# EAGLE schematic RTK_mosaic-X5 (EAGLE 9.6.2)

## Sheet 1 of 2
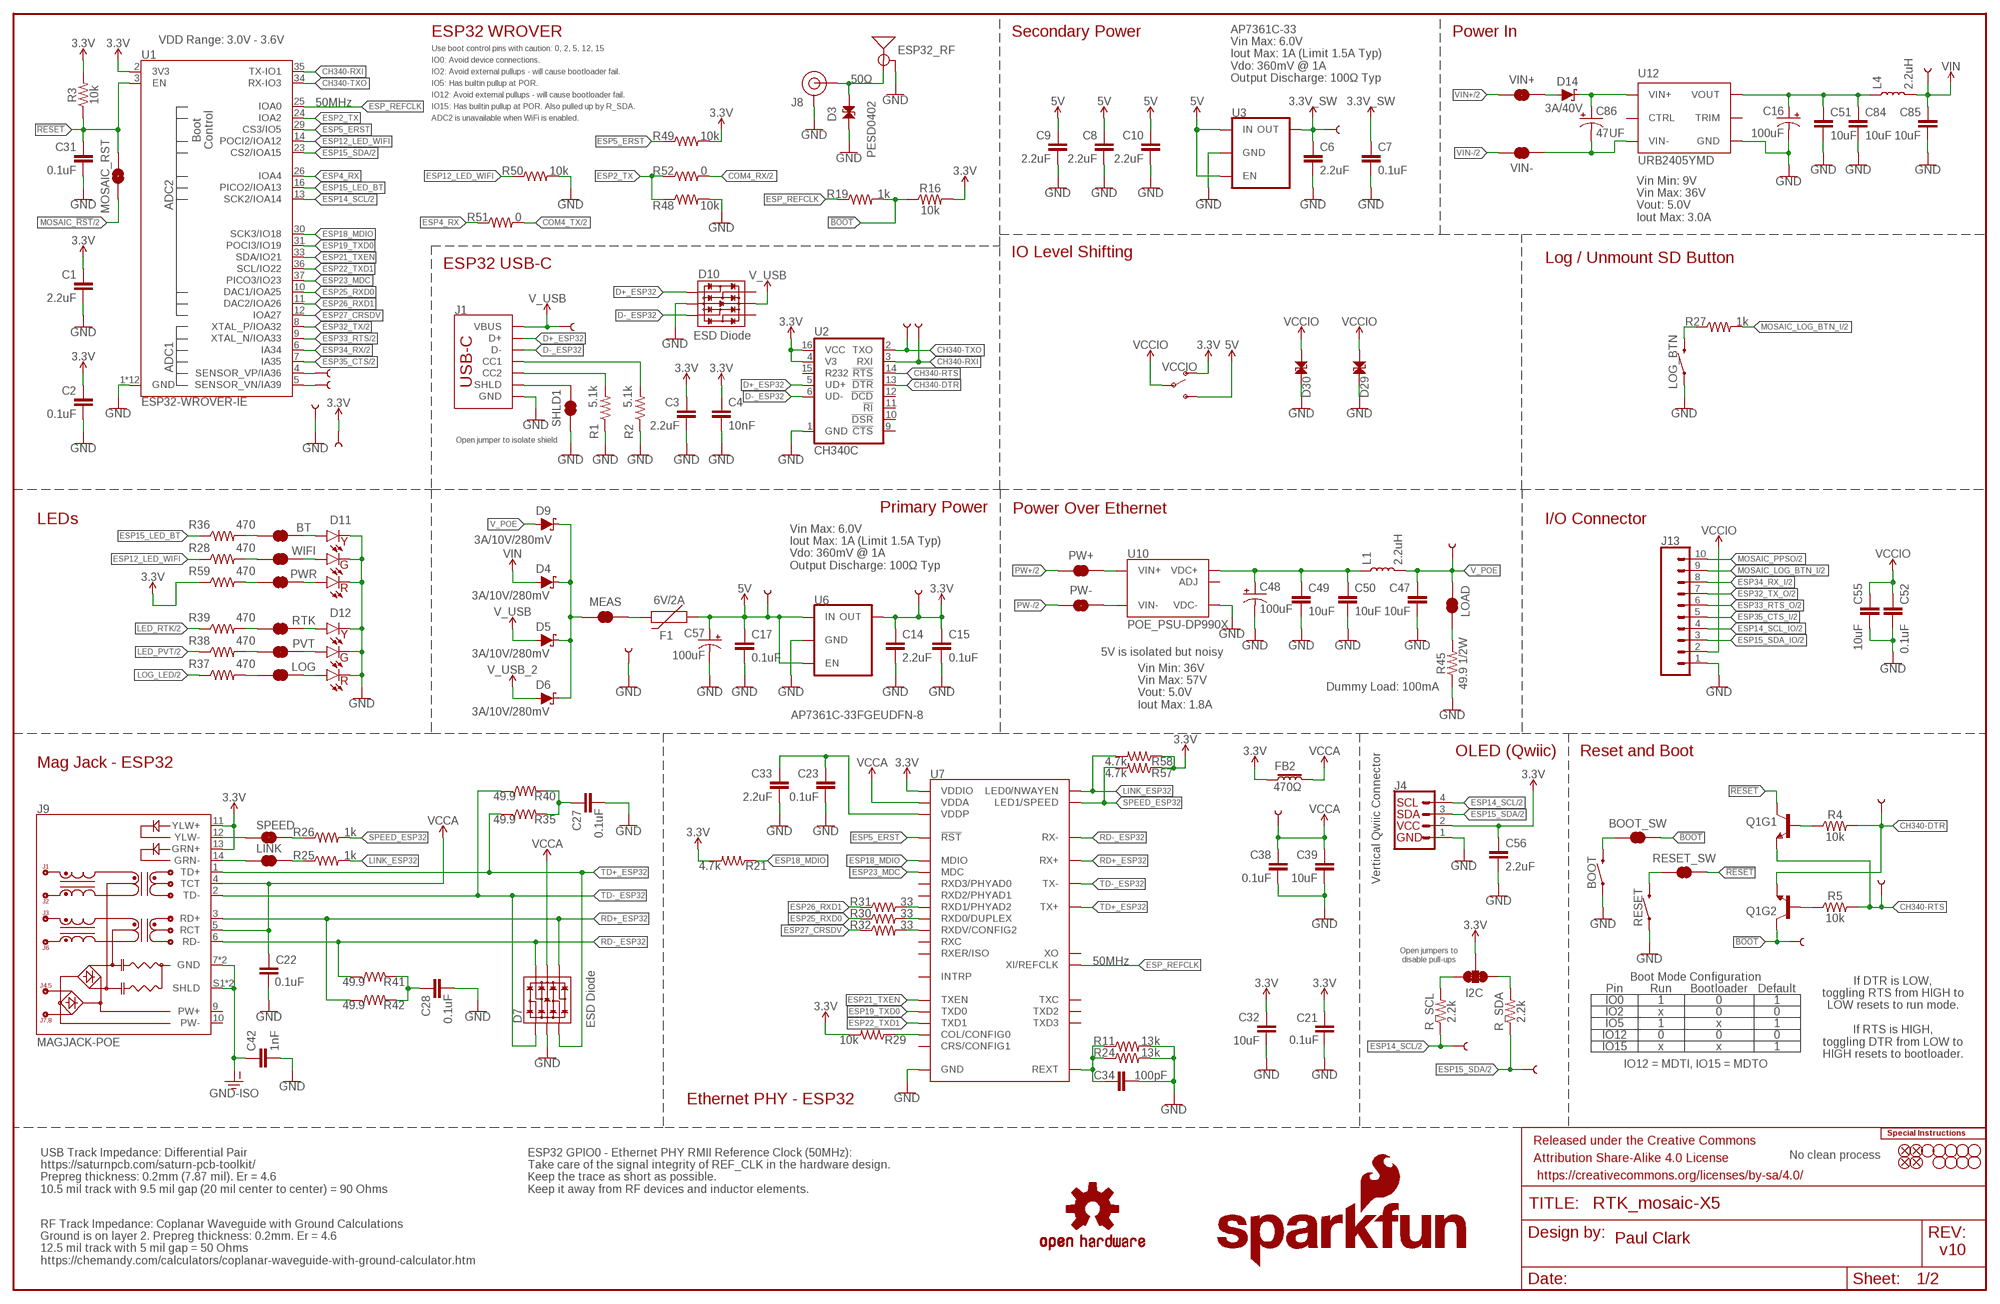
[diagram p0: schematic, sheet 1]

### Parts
3V3  TEST-POINTPOGO_PTH  [1X01_NO_SILK]
3V3_SW  TEST-POINTPOGO_PTH  [1X01_NO_SILK]
5V  TEST-POINTPOGO_PTH  [1X01_NO_SILK]
BOOT  MOMENTARY-SWITCH-SPST-PTH-RIGHT-ANGLE-8-020  [TACTILE_SWITCH_PTH_RA_8-020]
BOOT_SW  JUMPER-SMT_2_NC_TRACE_SILK  [SMT-JUMPER_2_NC_TRACE_SILK]
BT  JUMPER-SMT_2_NC_TRACE_SILK  [SMT-JUMPER_2_NC_TRACE_SILK]
C1  2.2uF  2.2UF-0603-10V-20%  [0603]
C2  0.1uF  0.1UF-0603-25V-5%  [0603]
C3  2.2uF  2.2UF-0603-10V-20%  [0603]
C4  10nF  10NF-0603-50V-10%  [0603]
C6  2.2uF  2.2UF-0603-10V-20%  [0603]
C7  0.1uF  0.1UF-0603-25V-5%  [0603]
C8  2.2uF  2.2UF-0603-10V-20%  [0603]
C9  2.2uF  2.2UF-0603-10V-20%  [0603]
C10  2.2uF  2.2UF-0603-10V-20%  [0603]
C14  2.2uF  2.2UF-0603-10V-20%  [0603]
C15  0.1uF  0.1UF-0603-25V-5%  [0603]
C16  100uF  100UF-POLAR-25V-20%(ELEC)  [PANASONIC_D]
C17  0.1uF  0.1UF-0603-25V-5%  [0603]
C21  0.1uF  0.1UF-0603-25V-5%  [0603]
C22  0.1uF  0.1UF-0603-25V-5%  [0603]
C23  0.1uF  0.1UF-0603-25V-5%  [0603]
C27  0.1uF  0.1UF-0603-25V-5%  [0603]
C28  0.1uF  0.1UF-0603-25V-5%  [0603]
C31  0.1uF  0.1UF-0603-25V-5%  [0603]
C32  10uF  10UF-0603-6.3V-20%  [0603]
C33  2.2uF  2.2UF-0603-10V-20%  [0603]
C34  100pF  100PF-0603-50V-5%  [0603]
C38  0.1uF  0.1UF-0603-25V-5%  [0603]
C39  10uF  10UF-0603-6.3V-20%  [0603]
C42  1nF  1.0NF/1000PF-1206-2KV-10%  [1206]
C47  10uF  10UF-0805-25V-10%  [0805]
C48  100uF  100UF-POLAR-25V-20%(ELEC)  [PANASONIC_D]
C49  10uF  10UF-0805-25V-10%  [0805]
C50  10uF  10UF-0805-25V-10%  [0805]
C51  10uF  10UF-0805-25V-10%  [0805]
C52  0.1uF  0.1UF-0603-25V-5%  [0603]
C55  10uF  10UF-0603-6.3V-20%  [0603]
C56  2.2uF  2.2UF-0603-10V-20%  [0603]
C57  100uF  100UF-POLAR-25V-20%(ELEC)  [PANASONIC_D]
C84  10uF  10UF-0805-25V-10%  [0805]
C85  10uF  10UF-0805-25V-10%  [0805]
C86  47UF  47UF-POLAR-PANASONIC_D-50V-20%  [PANASONIC_D]
D3  PESD0402  PESD0402-0402  [0402]
D4  3A/10V/280mV  DIODE-SCHOTTKY-BAT60A  [SOD-323]
D5  3A/10V/280mV  DIODE-SCHOTTKY-BAT60A  [SOD-323]
D6  3A/10V/280mV  DIODE-SCHOTTKY-BAT60A  [SOD-323]
D7  ESD Diode  TVS_DIODE_ARRAY_DT1042-04SO-7  [SOT-23-6]
D9  3A/10V/280mV  DIODE-SCHOTTKY-BAT60A  [SOD-323]
D10  ESD Diode  TVS_DIODE_ARRAY_DT1042-04SO-7  [SOT-23-6]
D11  Yellow Green Red  LED_TRIPLE-3MM_RIGHT-ANGLE_PTH_YELLOW_GREEN_RED  [CBI_LED_T-3MM_PTH]
D12  Yellow Green Red  LED_TRIPLE-3MM_RIGHT-ANGLE_PTH_YELLOW_GREEN_RED  [CBI_LED_T-3MM_PTH]
D14  3A/40V  DIODE-SCHOTTKY-B340A  [SMA-DIODE]
D29  PESD0402  PESD0402-0402  [0402]
D30  PESD0402  PESD0402-0402  [0402]
DTR  TEST-POINTPOGO_PTH  [1X01_NO_SILK]
ESP1  TEST-POINTPOGO_PTH  [1X01_NO_SILK]
ESP2  TEST-POINTPOGO_PTH  [1X01_NO_SILK]
ESP32_RF  ANTENNA-SMA-GROUNDEDEDGE_RPSMA  [RP-SMA-EDGE]
ESP36  TEST-POINTPOGO_PTH  [1X01_NO_SILK]
ESP39  TEST-POINTPOGO_PTH  [1X01_NO_SILK]
F1  6V/2A  PPTC_6V2A  [1210]
FB2  470Ω  FERRITE_BEAD-0603-470Ω-100MHZ-1A-200MILIΩ  [0603]
FD1  FIDUCIAL1X2  [FIDUCIAL-1X2]
FD2  FIDUCIAL1X2  [FIDUCIAL-1X2]
FD3  FIDUCIAL1X2  [FIDUCIAL-1X2]
FD4  FIDUCIAL1X2  [FIDUCIAL-1X2]
FRAME1  FRAME-LEDGER  [CREATIVE_COMMONS]
GND  TEST-POINTPOGO_PTH  [1X01_NO_SILK]
H1  STAND-OFFTIGHT  [STAND-OFF-TIGHT]
H2  STAND-OFFTIGHT  [STAND-OFF-TIGHT]
H3  STAND-OFFTIGHT  [STAND-OFF-TIGHT]
H4  STAND-OFFTIGHT  [STAND-OFF-TIGHT]
H5  STAND-OFFTIGHT  [STAND-OFF-TIGHT]
H6  STAND-OFFTIGHT  [STAND-OFF-TIGHT]
H7  STAND-OFFTIGHT  [STAND-OFF-TIGHT]
H8  STAND-OFFTIGHT  [STAND-OFF-TIGHT]
H10  STAND-OFFTIGHT  [STAND-OFF-TIGHT]
I2C  JUMPER-SMT_3_2-NC_TRACE_SILK  [SMT-JUMPER_3_2-NC_TRACE_SILK]
J1  USB_C_4-LAYER_PADS  [USB-C-16P_4LAYER-PADS]
J4  Vertical Qwiic Connector  QWIIC_CONNECTOR  [JST04_1MM_VERT]
J8  U.FL2PIN-REDUCED-FOOTPRINT  [U.FL_REDUCED_FOOTPRINT]
J9  MAGJACK-POE  [MAGJACK-SYM_LED]
J13  CONN_10_3.5MM_RA_HEADER  [1X10_SCREW_TERMINAL_3.5MM]
L1  2.2uH  INDUCTOR-0805_WIDE-2.2UH  [0805-WIDE]
L4  2.2uH  INDUCTOR-0805_WIDE-2.2UH  [0805-WIDE]
LINK  JUMPER-SMT_2_NC_TRACE_SILK  [SMT-JUMPER_2_NC_TRACE_SILK]
LOAD  JUMPER-SMT_2_NC_TRACE_SILK  [SMT-JUMPER_2_NC_TRACE_SILK]
LOG  JUMPER-SMT_2_NC_TRACE_SILK  [SMT-JUMPER_2_NC_TRACE_SILK]
LOG_BTN  MOMENTARY-SWITCH-SPST-PTH-RIGHT-ANGLE-8-020  [TACTILE_SWITCH_PTH_RA_8-020]
LOGO1  SPECIAL_INSTRUCTIONS-ORDERING  [ORDERING_INSTRUCTIONS]
LOGO4  OSHW-LOGOS  [OSHW-LOGO-S]
LOGO5  SFE_LOGO_NAME.2_INCH  [SFE_LOGO_NAME_.2]
LOGO6  SFE_LOGO_FLAME.2_INCH  [SFE_LOGO_FLAME_.2]
MEAS  JUMPER-COMBO_2_NC_TRACE  [COMBO-JUMPER_2_NC_TRACE]
MOSAIC_RST  JUMPER-COMBO_2_NO  [COMBO-JUMPER_2_NO]
PVT  JUMPER-SMT_2_NC_TRACE_SILK  [SMT-JUMPER_2_NC_TRACE_SILK]
PW+  JUMPER-COMBO_2_NC_TRACE  [COMBO-JUMPER_2_NC_TRACE]
PW-  JUMPER-COMBO_2_NC_TRACE  [COMBO-JUMPER_2_NC_TRACE]
PWR  JUMPER-SMT_2_NC_TRACE_SILK  [SMT-JUMPER_2_NC_TRACE_SILK]
Q1  TRANS_NPN_DUAL-MBT3904DW1T1  [SC70-6]
R1  5.1k  5.1KOHM5.1KOHM-0603-1/10W-1%  [0603]
R2  5.1k  5.1KOHM5.1KOHM-0603-1/10W-1%  [0603]
R3  10k  10KOHM-0603-1/10W-1%  [0603]
R4  10k  10KOHM-0603-1/10W-1%  [0603]
R5  10k  10KOHM-0603-1/10W-1%  [0603]
R11  13k  13KOHM-0603-1/10W-1%  [0603]
R16  10k  10KOHM-0603-1/10W-1%  [0603]
R19  1k  1KOHM-0603-1/10W-1%  [0603]
R21  4.7k  4.7KOHM-0603-1/10W-1%  [0603]
R24  13k  13KOHM-0603-1/10W-1%  [0603]
R25  1k  1KOHM-0603-1/10W-1%  [0603]
R26  1k  1KOHM-0603-1/10W-1%  [0603]
R27  1k  1KOHM-0603-1/10W-1%  [0603]
R28  470  470OHM-0603-1/10W-1%  [0603]
R29  10k  10KOHM-0603-1/10W-1%  [0603]
R30  33  33OHM-0603-1/10W-1%  [0603]
R31  33  33OHM-0603-1/10W-1%  [0603]
R32  33  33OHM-0603-1/10W-1%  [0603]
R35  49.9  49.9OHM-0603-1/10W-1%  [0603]
R36  470  470OHM-0603-1/10W-1%  [0603]
R37  470  470OHM-0603-1/10W-1%  [0603]
R38  470  470OHM-0603-1/10W-1%  [0603]
R39  470  470OHM-0603-1/10W-1%  [0603]
R40  49.9  49.9OHM-0603-1/10W-1%  [0603]
R41  49.9  49.9OHM-0603-1/10W-1%  [0603]
R42  49.9  49.9OHM-0603-1/10W-1%  [0603]
R45  49.9 1/2W  49.9OHM-1206-1/2W-1%  [1206]
R48  10k  10KOHM-0603-1/10W-1%  [0603]
R49  10k  10KOHM-0603-1/10W-1%  [0603]
R50  10k  10KOHM-0603-1/10W-1%  [0603]
R51  0  0OHM-0603-1/10W  [0603]
R52  0  0OHM-0603-1/10W  [0603]
R57  4.7k  4.7KOHM-0603-1/10W-1%  [0603]
R58  4.7k  4.7KOHM-0603-1/10W-1%  [0603]
R59  470  470OHM-0603-1/10W-1%  [0603]
R_SCL  2.2k  2.2KOHM-0603-1/10W-1%  [0603]
R_SDA  2.2k  2.2KOHM-0603-1/10W-1%  [0603]
RESET  MOMENTARY-SWITCH-SPST-PTH-RIGHT-ANGLE-8-020  [TACTILE_SWITCH_PTH_RA_8-020]
RESET_SW  JUMPER-SMT_2_NC_TRACE_SILK  [SMT-JUMPER_2_NC_TRACE_SILK]
RTK  JUMPER-SMT_2_NC_TRACE_SILK  [SMT-JUMPER_2_NC_TRACE_SILK]
RTS  TEST-POINTPOGO_PTH  [1X01_NO_SILK]
RX  TEST-POINTPOGO_PTH  [1X01_NO_SILK]
SCL2  TEST-POINTPOGO_PTH  [1X01_NO_SILK]
SDA2  TEST-POINTPOGO_PTH  [1X01_NO_SILK]
SHLD1  JUMPER-SMT_2_NC_TRACE_SILK  [SMT-JUMPER_2_NC_TRACE_SILK]
SPEED  JUMPER-SMT_2_NC_TRACE_SILK  [SMT-JUMPER_2_NC_TRACE_SILK]
TP_BOOT  TEST-POINTPOGO_PTH  [1X01_NO_SILK]
TX  TEST-POINTPOGO_PTH  [1X01_NO_SILK]
U1  ESP32-WROVER-IE  ESP32-WROVER-E/IE_IE-N16R8  [ESP32-WROVER-E/IE]
U2  CH340C  [SO016]
U3  AP7361C-33FGEUDFN-8  [UDFN-8]
U6  AP7361C-33FGEUDFN-8  [UDFN-8]
U7  KSZ8041NLI  KSZ8041NL  [MLF55Q-32LD]
U10  POE_PSU-DP990X  [DP990X]
U12  URB2405YMD  URB_YMD-15WR3__URB2405YMD-15WR3  [URB_YMD-15WR3]
VCCA  TEST-POINTPOGO_PTH  [1X01_NO_SILK]
VCCIO  SWITCH-SPDT-SMD-AYZ0202  [SWITCH_DPDT_SMD_AYZ0202]
VIN  TEST-POINTPOGO_PTH  [1X01_NO_SILK]
VIN+  JUMPER-COMBO_2_NC_TRACE  [COMBO-JUMPER_2_NC_TRACE]
VIN-  JUMPER-COMBO_2_NC_TRACE  [COMBO-JUMPER_2_NC_TRACE]
VPOE  TEST-POINTPOGO_PTH  [1X01_NO_SILK]
VUSB  TEST-POINTPOGO_PTH  [1X01_NO_SILK]
WIFI  JUMPER-SMT_2_NC_TRACE_SILK  [SMT-JUMPER_2_NC_TRACE_SILK]

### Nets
3.3V: 3V3.1 C1.1 C2.1 C3.1 C4.1 C14.1 C15.1 C21.1 C32.1 C56.1 ESP2.1 FB2.1 I2C.2 J4.2 J9.11(YLW+) J9.13(GRN+) R3.2 R16.2 R21.2 R29.2 R49.2 R57.1 R58.1 R59.1 U1.2(3V3) U2.4(V3) U2.16(VCC) U6.1(OUT) U7.17(VDDIO) VCCIO.1(O) ; also sheet 2
3.3V_SW: 3V3_SW.1 C6.1 C7.1 U3.1(OUT) ; also sheet 2
5V: 5V.1 C8.1 C9.1 C10.1 C17.1 C57.+ F1.1 U3.5(EN) U3.8(IN) U6.5(EN) U6.8(IN) VCCIO.3(S) ; also sheet 2
5V_RAW: C48.+ C49.1 C50.1 L1.1 U10.1(VDC+) U10.2(VDC+)
5V_RAW1: C16.+ C51.1 C84.1 L4.1 U12.4(VOUT)
!BOOT!: BOOT_SW.1 Q1.6(C) R16.1 R19.2 TP_BOOT.1
!RESET!: C31.1 MOSAIC_RST.2 MOSAIC_RST.4 Q1.3(C) R3.1 RESET_SW.1 U1.3(EN)
CH340-DTR: DTR.1 Q1.1(E) R4.2 U2.13(!DTR)
CH340-RTS: Q1.4(E) R5.2 RTS.1 U2.14(!RTS)
CH340-RXI: TX.1 U1.35(TX-IO1) U2.3(RXI)
CH340-TXO: RX.1 U1.34(RX-IO3) U2.2(TXO)
COM4_RX: R52.2 ; also sheet 2
COM4_TX: R51.2 ; also sheet 2
D+_ESP32: D10.1(IO1) J1.A6(D+) J1.B6(D+) U2.5(UD+)
D-_ESP32: D10.3(IO2) J1.A7(D-) J1.B7(D-) U2.6(UD-)
ESP2_TX: R48.1 R52.1 U1.24(IOA2)
ESP4_RX: R51.1 U1.26(IOA4)
ESP5_ERST: R49.1 U1.29(CS3/IO5) U7.32(!RST!)
ESP12_LED_WIFI: R28.1 R50.1 U1.14(POCI2/IOA12)
ESP14_SCL: J4.4 R_SCL.1 SCL2.1 U1.13(SCK2/IOA14) ; also sheet 2
ESP14_SCL_IO: J13.4 ; also sheet 2
ESP15_LED_BT: R36.1 U1.16(PICO2/IOA13)
ESP15_SDA: J4.3 R_SDA.1 SDA2.1 U1.23(CS2/IOA15) ; also sheet 2
ESP15_SDA_IO: J13.3 ; also sheet 2
ESP18_MDIO: R21.1 U1.30(SCK3/IO18) U7.11(MDIO)
ESP19_TXD0: U1.31(POCI3/IO19) U7.24(TXD0)
ESP21_TXEN: U1.33(SDA/IO21) U7.23(TXEN)
ESP22_TXD1: U1.36(SCL/IO22) U7.25(TXD1)
ESP23_MDC: U1.37(PICO3/IO23) U7.12(MDC)
ESP25_RXD0: R30.1 U1.10(DAC1/IOA25)
ESP26_RXD1: R31.1 U1.11(DAC2/IOA26)
ESP27_CRSDV: R32.1 U1.12(IOA27)
ESP32_RF: D3.1 ESP32_RF.SIG(SIGNAL) J8.FEED(SIGNAL)
ESP32_TX: U1.8(XTAL_P/IOA32) ; also sheet 2
ESP32_TX_O: J13.7 ; also sheet 2
ESP33_RTS: U1.9(XTAL_N/IOA33) ; also sheet 2
ESP33_RTS_O: J13.6 ; also sheet 2
ESP34_RX: U1.6(IA34) ; also sheet 2
ESP34_RX_I: J13.8 ; also sheet 2
ESP35_CTS: U1.7(IA35) ; also sheet 2
ESP35_CTS_I: J13.5 ; also sheet 2
ESP36: ESP36.1 U1.4(SENSOR_VP/IA36)
ESP39: ESP39.1 U1.5(SENSOR_VN/IA39)
ESP_REFCLK: R19.1 U1.25(IOA0) U7.9(XI/REFCLK)
GND: BOOT.1 C1.2 C2.2 C3.2 C4.2 C6.2 C7.2 C8.2 C9.2 C10.2 C14.2 C15.2 C16.- C17.2 C21.2 C22.2 C23.2 C27.2 C28.2 C31.2 C32.2 C33.2 C34.2 C38.2 C39.2 C42.2 C47.2 C48.- C49.2 C50.2 C51.2 C52.2 C55.2 C56.2 C57.- C84.2 C85.2 D3.2 D7.2(VSS) D10.2(VSS) D11.CATHODE_1(YELLOW_CATHODE) D11.CATHODE_2(GREEN_CATHODE) D11.CATHODE_3(RED_CATHODE) D12.CATHODE_1(YELLOW_CATHODE) D12.CATHODE_2(GREEN_CATHODE) D12.CATHODE_3(RED_CATHODE) D29.2 D30.2 ESP1.1 ESP32_RF.GND@0(GND) ESP32_RF.GND@1(GND) ESP32_RF.GND@2(GND) ESP32_RF.GND@3(GND) GND.1 J1.GND J1.GND2(GND) J4.1 J8.1(GND) J8.2(GND) J13.1 LOG_BTN.1 R1.1 R2.1 R11.2 R24.2 R45.1 R48.2 R50.2 RESET.1 SHLD1.1 U1.1(GND) U1.15(GND) U1.38(GND) U1.GND U1.GNDT1(GND) U1.GNDT2(GND) U1.GNDT3(GND) U1.GNDT4(GND) U1.GNDT5(GND) U1.GNDT6(GND) U1.GNDT7(GND) U1.GNDT8(GND) U2.1(GND) U3.4(GND) U3.EP(GND) U6.4(GND) U6.EP(GND) U7.1(GND) U7.GND U10.3(VDC-) U12.6(GND) ; also sheet 2
GND-ISO: C42.1 J9.7(GND) J9.8(GND) J9.S1(SHLD) J9.S2(SHLD) ; also sheet 2
LED_PVT: R38.1 ; also sheet 2
LED_RTK: R39.1 ; also sheet 2
LINK_ESP32: R25.2 R58.2 U7.30(LED0/NWAYEN)
LOG_LED: R37.1 ; also sheet 2
MEAS: D4.C D5.C D6.C D9.C MEAS.2 MEAS.4
MOSAIC_!RST!: MOSAIC_RST.1 MOSAIC_RST.3 ; also sheet 2
MOSAIC_LOG_BTN_I: J13.9 R27.2 ; also sheet 2
MOSAIC_PPSO: J13.10 ; also sheet 2
N$1: J1.B5(CC2) R1.2
N$2: J1.A5(CC1) R2.2
N$3: J9.14(GRN-) LINK.1
N$4: Q1.2(B) R5.1
N$5: Q1.5(B) R4.1
N$7: J9.12(YLW-) SPEED.1
N$10: F1.2 MEAS.1 MEAS.3
N$11: LOG_BTN.2 R27.1
N$12: R26.1 SPEED.2
N$14: I2C.3 R_SCL.2
N$15: I2C.1 R_SDA.2
N$16: LOG.2 R37.2
N$17: D12.ANODE_3(RED_ANODE) LOG.1
N$18: D11.ANODE_2(GREEN_ANODE) WIFI.1
N$19: C27.1 R35.2 R40.2
N$20: C28.1 R41.2 R42.2
N$21: LINK.2 R25.1
N$22: BT.1 D11.ANODE_1(YELLOW_ANODE)
N$23: C23.1 C33.1 U7.2(VDDP)
N$24: C34.1 R11.1 R24.1 U7.10(REXT)
N$25: R29.1 U7.28(COL/CONFIG0)
N$26: BT.2 R36.2
N$27: LOAD.1 R45.2
N$28: RESET.2 RESET_SW.2
N$29: BOOT.2 BOOT_SW.2
N$30: R30.2 U7.16(RXD0/DUPLEX)
N$31: R31.2 U7.15(RXD1/PHYAD2)
N$32: R28.2 WIFI.2
N$35: D12.ANODE_2(GREEN_ANODE) PVT.1
N$36: D12.ANODE_1(YELLOW_ANODE) RTK.1
N$37: R39.2 RTK.2
N$38: PVT.2 R38.2
N$39: R32.2 U7.18(RXDV/CONFIG2)
N$44: PWR.2 R59.2
N$45: D11.ANODE_3(RED_ANODE) PWR.1
PW1+: PW+.1 PW+.3 U10.5(VIN+) U10.6(VIN+)
PW1-: PW-.1 PW-.3 U10.7(VIN-) U10.8(VIN-)
PW+: PW+.2 PW+.4 ; also sheet 2
PW-: PW-.2 PW-.4 ; also sheet 2
RD+_ESP32: D7.4(IO3) J9.3(RD+) R42.1 U7.5(RX+)
RD-_ESP32: D7.6(IO4) J9.6(RD-) R41.1 U7.4(RX-)
SHIELD: J1.SHLD1(SHLD) J1.SHLD2(SHLD) J1.SHLD3(SHLD) J1.SHLD4(SHLD) SHLD1.2
SPEED_ESP32: R26.2 R57.2 U7.31(LED1/SPEED)
TD+_ESP32: D7.3(IO2) J9.1(TD+) R35.1 U7.7(TX+)
TD-_ESP32: D7.1(IO1) J9.2(TD-) R40.1 U7.6(TX-)
V_POE: C47.1 D9.A L1.2 LOAD.2 VPOE.1
V_USB: D5.A D10.5(VCC) J1.VBUS1(VBUS) J1.VBUS2(VBUS) VUSB.1
V_USB_2: D6.A ; also sheet 2
VCCA: C22.1 C38.1 C39.1 D7.5(VCC) FB2.2 J9.4(TCT) J9.5(RCT) U7.3(VDDA) VCCA.1
VCCIO: C52.1 C55.1 D29.1 D30.1 J13.2 VCCIO.2(P) ; also sheet 2
VIN: C85.1 D4.A L4.2 VIN.1
VIN1+: D14.A VIN+.1 VIN+.3
VIN1-: C86.- U12.2(VIN-) VIN-.2 VIN-.4
VIN2+: C86.+ D14.C U12.3(VIN+)
VIN+: VIN+.2 VIN+.4 ; also sheet 2
VIN-: VIN-.1 VIN-.3 ; also sheet 2
Unconnected: D10.4(IO3) D10.6(IO4) J9.9(PW+) J9.10(PW-) U2.9(!CTS) U2.10(!DSR) U2.11(!RI) U2.12(!DCD) U2.15(R232) U7.8(XO) U7.13(RXD3/PHYAD0) U7.14(RXD2/PHYAD1) U7.19(RXC) U7.20(RXER/ISO) U7.21(INTRP) U7.22(TXC) U7.26(TXD2) U7.27(TXD3) U7.29(CRS/CONFIG1) U10.4(ADJ) U12.1(CTRL) U12.5(TRIM)

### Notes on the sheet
- Secondary Power | Power In
- VDD Range: 3.0V - 3.6V | ESP32 WROVER
- Use boot control pins with caution: 0, 2, 5, 12, 15
- IO0: Avoid device connections.
- IO2: Avoid external pullups - will cause bootloader fail.
- AP7361C-33
  Vin Max: 6.0V
  Iout Max: 1A (Limit 1.5A Typ)
  Vdo: 360mV @ 1A
  Output Discharge: 100Ω Typ
- IO5: Has builtin pullup at POR. | 50Ω
- IO12: Avoid external pullups - will cause bootloader fail.
- 50MHz | IO15: Has builtin pullup at POR. Also pulled up by R_SDA.
- ADC2 is unavailable when WiFi is enabled.
- Vin Min: 9V
  Vin Max: 36V
  Vout: 5.0V
  Iout Max: 3.0A
- IO Level Shifting
- Log / Unmount SD Button
- ESP32 USB-C
- Open jumper to isolate shield
- Primary Power | Power Over Ethernet
- LEDs | I/O Connector
- Vin Max: 6.0V
  Iout Max: 1A (Limit 1.5A Typ)
  Vdo: 360mV @ 1A
  Output Discharge: 100Ω Typ
- 5V is isolated but noisy
- Dummy Load: 100mA
- Vin Min: 36V
  Vin Max: 57V
  Vout: 5.0V
  Iout Max: 1.8A
- OLED (Qwiic) | Reset and Boot
- Mag Jack - ESP32
- Open jumpers to
  disable pull-ups
- 50MHz
- Boot Mode Configuration
- If DTR is LOW,
  toggling RTS from HIGH to
  LOW resets to run mode.
  
  If RTS is HIGH,
  toggling DTR from LOW to
  HIGH resets to bootloader.
- Pin | Run | Bootloader | Default
- IO0 | 1 | 0 | 1
- IO2 | x | 0 | 0
- IO5 | 1 | x | 1
- IO12 | 0 | 0 | 0
- IO15 | x | x | 1
- IO12 = MDTI, IO15 = MDTO
- Ethernet PHY - ESP32
- USB Track Impedance: Differential Pair
  https://saturnpcb.com/saturn-pcb-toolkit/
  Prepreg thickness: 0.2mm (7.87 mil). Er = 4.6
  10.5 mil track with 9.5 mil gap (20 mil center to center) = 90 Ohms
- ESP32 GPIO0 - Ethernet PHY RMII Reference Clock (50MHz):
  Take care of the signal integrity of REF_CLK in the hardware design.
  Keep the trace as short as possible.
  Keep it away from RF devices and inductor elements.
- No clean process
- Paul Clark
- v10
- RF Track Impedance: Coplanar Waveguide with Ground Calculations
  Ground is on layer 2. Prepreg thickness: 0.2mm. Er = 4.6
  12.5 mil track with 5 mil gap = 50 Ohms
  https://chemandy.com/calculators/coplanar-waveguide-with-ground-calculator.htm

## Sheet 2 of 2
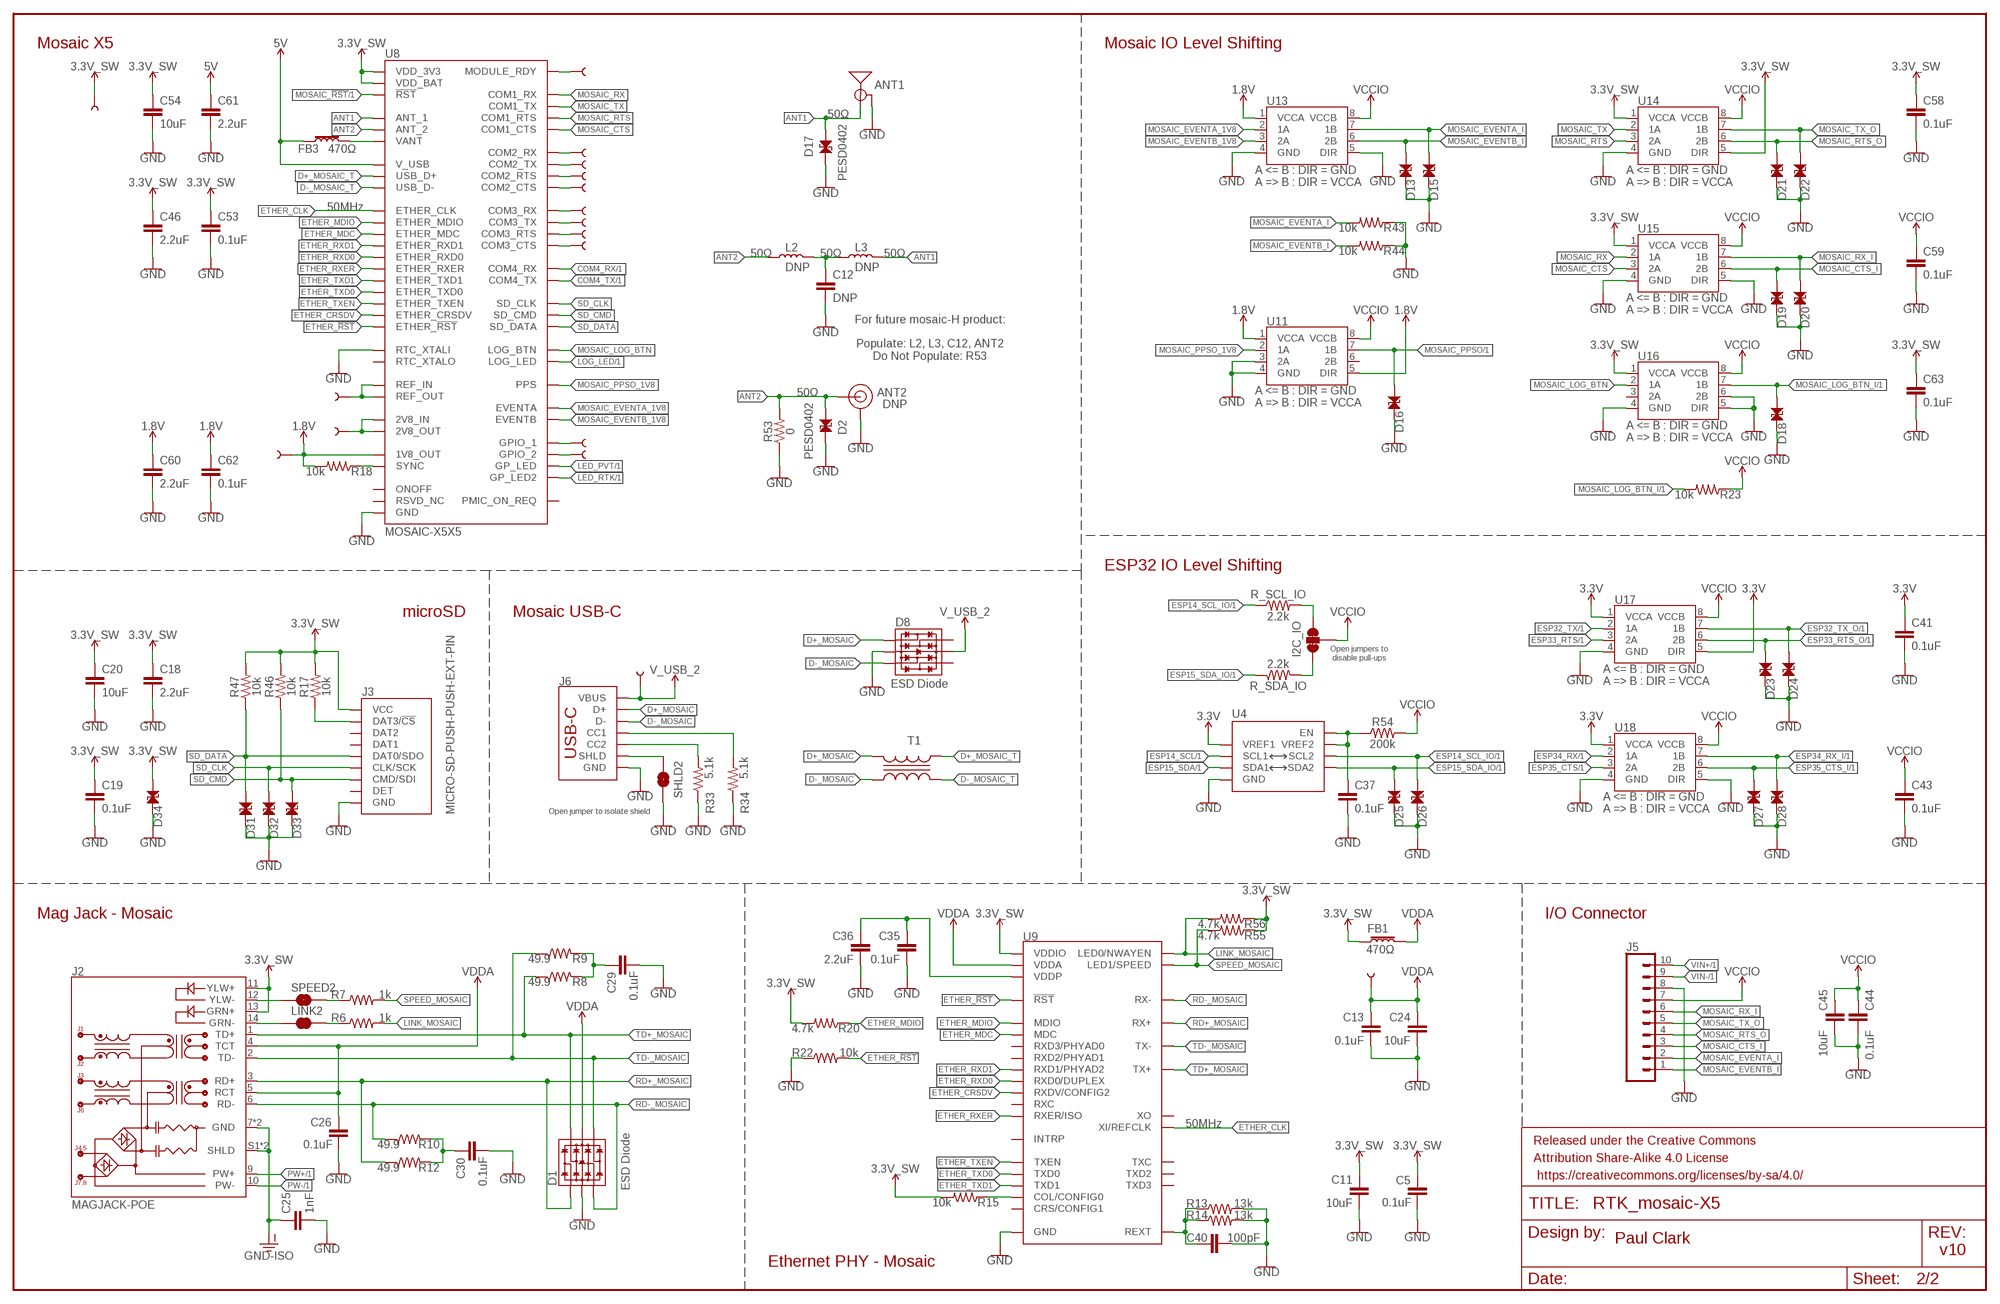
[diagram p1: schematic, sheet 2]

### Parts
1V8  TEST-POINTPOGO_PTH  [1X01_NO_SILK]
2V8  TEST-POINTPOGO_PTH  [1X01_NO_SILK]
ANT1  ANTENNA-SMA-GROUNDEDEDGE_SMA  [SMA-EDGE]
ANT2  DNP  U.FL2PIN-REDUCED__DNP_NO_CREAM  [U.FL_REDUCED_FOOTPRINT__NO_CREAM]
C5  0.1uF  0.1UF-0603-25V-5%  [0603]
C11  10uF  10UF-0603-6.3V-20%  [0603]
C12  DNP  DNP-0603_NO_CREAM  [0603_NO_CREAM]
C13  0.1uF  0.1UF-0603-25V-5%  [0603]
C18  2.2uF  2.2UF-0603-10V-20%  [0603]
C19  0.1uF  0.1UF-0603-25V-5%  [0603]
C20  10uF  10UF-0603-6.3V-20%  [0603]
C24  10uF  10UF-0603-6.3V-20%  [0603]
C25  1nF  1.0NF/1000PF-1206-2KV-10%  [1206]
C26  0.1uF  0.1UF-0603-25V-5%  [0603]
C29  0.1uF  0.1UF-0603-25V-5%  [0603]
C30  0.1uF  0.1UF-0603-25V-5%  [0603]
C35  0.1uF  0.1UF-0603-25V-5%  [0603]
C36  2.2uF  2.2UF-0603-10V-20%  [0603]
C37  0.1uF  0.1UF-0603-25V-5%  [0603]
C40  100pF  100PF-0603-50V-5%  [0603]
C41  0.1uF  0.1UF-0603-25V-5%  [0603]
C43  0.1uF  0.1UF-0603-25V-5%  [0603]
C44  0.1uF  0.1UF-0603-25V-5%  [0603]
C45  10uF  10UF-0603-6.3V-20%  [0603]
C46  2.2uF  2.2UF-0603-10V-20%  [0603]
C53  0.1uF  0.1UF-0603-25V-5%  [0603]
C54  10uF  10UF-0603-6.3V-20%  [0603]
C58  0.1uF  0.1UF-0603-25V-5%  [0603]
C59  0.1uF  0.1UF-0603-25V-5%  [0603]
C60  2.2uF  2.2UF-0603-10V-20%  [0603]
C61  2.2uF  2.2UF-0603-10V-20%  [0603]
C62  0.1uF  0.1UF-0603-25V-5%  [0603]
C63  0.1uF  0.1UF-0603-25V-5%  [0603]
COM2_CTS  TEST-POINTPOGO_PTH  [1X01_NO_SILK]
COM2_RTS  TEST-POINTPOGO_PTH  [1X01_NO_SILK]
COM2_RX  TEST-POINTPOGO_PTH  [1X01_NO_SILK]
COM2_TX  TEST-POINTPOGO_PTH  [1X01_NO_SILK]
COM3_CTS  TEST-POINTPOGO_PTH  [1X01_NO_SILK]
COM3_RTS  TEST-POINTPOGO_PTH  [1X01_NO_SILK]
COM3_RX  TEST-POINTPOGO_PTH  [1X01_NO_SILK]
COM3_TX  TEST-POINTPOGO_PTH  [1X01_NO_SILK]
D1  ESD Diode  TVS_DIODE_ARRAY_DT1042-04SO-7  [SOT-23-6]
D2  PESD0402  PESD0402-0402  [0402]
D8  ESD Diode  TVS_DIODE_ARRAY_DT1042-04SO-7  [SOT-23-6]
D13  PESD0402  PESD0402-0402  [0402]
D15  PESD0402  PESD0402-0402  [0402]
D16  PESD0402  PESD0402-0402  [0402]
D17  PESD0402  PESD0402-0402  [0402]
D18  PESD0402  PESD0402-0402  [0402]
D19  PESD0402  PESD0402-0402  [0402]
D20  PESD0402  PESD0402-0402  [0402]
D21  PESD0402  PESD0402-0402  [0402]
D22  PESD0402  PESD0402-0402  [0402]
D23  PESD0402  PESD0402-0402  [0402]
D24  PESD0402  PESD0402-0402  [0402]
D25  PESD0402  PESD0402-0402  [0402]
D26  PESD0402  PESD0402-0402  [0402]
D27  PESD0402  PESD0402-0402  [0402]
D28  PESD0402  PESD0402-0402  [0402]
D31  PESD0402  PESD0402-0402  [0402]
D32  PESD0402  PESD0402-0402  [0402]
D33  PESD0402  PESD0402-0402  [0402]
D34  PESD0402  PESD0402-0402  [0402]
FB1  470Ω  FERRITE_BEAD-0603-470Ω-100MHZ-1A-200MILIΩ  [0603]
FB3  470Ω  FERRITE_BEAD-0603-470Ω-100MHZ-1A-200MILIΩ  [0603]
FRAME3  FRAME-LEDGERNO_FOOTPRINT  [DUMMY]
GPIO_1  TEST-POINTPOGO_PTH  [1X01_NO_SILK]
GPIO_2  TEST-POINTPOGO_PTH  [1X01_NO_SILK]
I2C_IO  JUMPER-SMT_3_2-NC_TRACE_SILK  [SMT-JUMPER_3_2-NC_TRACE_SILK]
J2  MAGJACK-POE  [MAGJACK-SYM_LED]
J3  MICRO-SD-PUSH-PUSH-EXT-PIN  [MICROSD-EXTERNALPIN]
J5  CONN_10_3.5MM_RA_HEADER  [1X10_SCREW_TERMINAL_3.5MM]
J6  USB_C_4-LAYER_PADS  [USB-C-16P_4LAYER-PADS]
L2  DNP  DNP-0603_NO-CREAM  [0603_NO-CREAM]
L3  DNP  DNP-0603_NO-CREAM  [0603_NO-CREAM]
LINK2  JUMPER-SMT_2_NC_TRACE_SILK  [SMT-JUMPER_2_NC_TRACE_SILK]
R6  1k  1KOHM-0603-1/10W-1%  [0603]
R7  1k  1KOHM-0603-1/10W-1%  [0603]
R8  49.9  49.9OHM-0603-1/10W-1%  [0603]
R9  49.9  49.9OHM-0603-1/10W-1%  [0603]
R10  49.9  49.9OHM-0603-1/10W-1%  [0603]
R12  49.9  49.9OHM-0603-1/10W-1%  [0603]
R13  13k  13KOHM-0603-1/10W-1%  [0603]
R14  13k  13KOHM-0603-1/10W-1%  [0603]
R15  10k  10KOHM-0603-1/10W-1%  [0603]
R17  10k  10KOHM-0603-1/10W-1%  [0603]
R18  10k  10KOHM-0603-1/10W-1%  [0603]
R20  4.7k  4.7KOHM-0603-1/10W-1%  [0603]
R22  10k  10KOHM-0603-1/10W-1%  [0603]
R23  10k  10KOHM-0603-1/10W-1%  [0603]
R33  5.1k  5.1KOHM5.1KOHM-0603-1/10W-1%  [0603]
R34  5.1k  5.1KOHM5.1KOHM-0603-1/10W-1%  [0603]
R43  10k  10KOHM-0603-1/10W-1%  [0603]
R44  10k  10KOHM-0603-1/10W-1%  [0603]
R46  10k  10KOHM-0603-1/10W-1%  [0603]
R47  10k  10KOHM-0603-1/10W-1%  [0603]
R53  0  0OHM-0603-1/10W  [0603]
R54  200k  200KOHM-0603-1/10W-1%  [0603]
R55  4.7k  4.7KOHM-0603-1/10W-1%  [0603]
R56  4.7k  4.7KOHM-0603-1/10W-1%  [0603]
R_SCL_IO  2.2k  2.2KOHM-0603-1/10W-1%  [0603]
R_SDA_IO  2.2k  2.2KOHM-0603-1/10W-1%  [0603]
RDY  TEST-POINTPOGO_PTH  [1X01_NO_SILK]
RDY1  TEST-POINTPOGO_PTH  [1X01_NO_SILK]
REF  TEST-POINTPOGO_PTH  [1X01_NO_SILK]
SHLD2  JUMPER-SMT_2_NC_TRACE_SILK  [SMT-JUMPER_2_NC_TRACE_SILK]
SPEED2  JUMPER-SMT_2_NC_TRACE_SILK  [SMT-JUMPER_2_NC_TRACE_SILK]
T1  TRANSFORMER0508  [RFCMF1220100M4T]
U4  PCA9306VSSOP_8PIN  [VSSOP_8PIN]
U8  MOSAIC-X5X5  [MOSAIC_LGA]
U9  KSZ8041NLI  KSZ8041NL  [MLF55Q-32LD]
U11  74LVC2T45DC  [VSSOP8_(SOT765-1)]
U13  74LVC2T45DC  [VSSOP8_(SOT765-1)]
U14  74LVC2T45DC  [VSSOP8_(SOT765-1)]
U15  74LVC2T45DC  [VSSOP8_(SOT765-1)]
U16  74LVC2T45DC  [VSSOP8_(SOT765-1)]
U17  74LVC2T45DC  [VSSOP8_(SOT765-1)]
U18  74LVC2T45DC  [VSSOP8_(SOT765-1)]
VDDA  TEST-POINTPOGO_PTH  [1X01_NO_SILK]
VUSB2  TEST-POINTPOGO_PTH  [1X01_NO_SILK]

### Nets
1.8V: 1V8.1 C60.1 C62.1 R18.2 U8.AC4(1V8_OUT) U11.1(VCCA) U11.5(DIR) U13.1(VCCA)
2V8: 2V8.1 U8.M23(2V8_IN) U8.N23(2V8_OUT)
3.3V: C41.1 U4.P2(VREF1) U17.1(VCCA) U17.5(DIR) U18.1(VCCA) ; also sheet 1
3.3V_SW: C5.1 C11.1 C18.1 C19.1 C20.1 C46.1 C53.1 C54.1 C58.1 C63.1 D34.1 FB1.1 J2.11(YLW+) J2.13(GRN+) J3.4(VCC) R15.2 R17.2 R20.2 R46.2 R47.2 R55.1 R56.1 RDY1.1 U8.A18(VDD_3V3) U8.A19(VDD_3V3) U8.A20(VDD_3V3) U8.B8(VDD_BAT) U8.B18(VDD_3V3) U8.B19(VDD_3V3) U8.B20(VDD_3V3) U8.C18(VDD_3V3) U8.C19(VDD_3V3) U8.C20(VDD_3V3) U9.17(VDDIO) U14.1(VCCA) U14.5(DIR) U15.1(VCCA) U16.1(VCCA) ; also sheet 1
5V: C61.1 FB3.1 U8.A8(V_USB) ; also sheet 1
ANT1: ANT1.SIG(SIGNAL) D17.1 L3.2 U8.AC20(ANT_1)
ANT2: ANT2.FEED(SIGNAL) D2.1 L2.1 R53.2 U8.V23(ANT_2)
COM2_CTS: COM2_CTS.1 U8.J1(COM2_CTS)
COM2_RTS: COM2_RTS.1 U8.G1(COM2_RTS)
COM2_RX: COM2_RX.1 U8.F1(COM2_RX)
COM2_TX: COM2_TX.1 U8.H1(COM2_TX)
COM3_CTS: COM3_CTS.1 U8.N1(COM3_CTS)
COM3_RTS: COM3_RTS.1 U8.L1(COM3_RTS)
COM3_RX: COM3_RX.1 U8.K1(COM3_RX)
COM3_TX: COM3_TX.1 U8.M1(COM3_TX)
COM4_RX: U8.D3(COM4_RX) ; also sheet 1
COM4_TX: U8.E3(COM4_TX) ; also sheet 1
D+_MOSAIC: D8.1(IO1) J6.A6(D+) J6.B6(D+) T1.A2
D+_MOSAIC_T: T1.A1 U8.A5(USB_D+)
D-_MOSAIC: D8.3(IO2) J6.A7(D-) J6.B7(D-) T1.B2
D-_MOSAIC_T: T1.B1 U8.A6(USB_D-)
ESP14_SCL: U4.P3(SCL1) ; also sheet 1
ESP14_SCL_IO: D26.1 R_SCL_IO.1 U4.P6(SCL2) ; also sheet 1
ESP15_SDA: U4.P4(SDA1) ; also sheet 1
ESP15_SDA_IO: D25.1 R_SDA_IO.1 U4.P5(SDA2) ; also sheet 1
ESP32_TX: U17.2(1A) ; also sheet 1
ESP32_TX_O: D24.1 U17.7(1B) ; also sheet 1
ESP33_RTS: U17.3(2A) ; also sheet 1
ESP33_RTS_O: D23.1 U17.6(2B) ; also sheet 1
ESP34_RX: U18.2(1A) ; also sheet 1
ESP34_RX_I: D28.1 U18.7(1B) ; also sheet 1
ESP35_CTS: U18.3(2A) ; also sheet 1
ESP35_CTS_I: D27.1 U18.6(2B) ; also sheet 1
ETHER_!RST!: R22.2 U8.F2(ETHER_!RST!) U9.32(!RST!)
ETHER_CLK: U8.AA2(ETHER_CLK) U9.9(XI/REFCLK)
ETHER_CRSDV: U8.N2(ETHER_CRSDV) U9.18(RXDV/CONFIG2)
ETHER_MDC: U8.V2(ETHER_MDC) U9.12(MDC)
ETHER_MDIO: R20.1 U8.W2(ETHER_MDIO) U9.11(MDIO)
ETHER_RXD0: U8.R2(ETHER_RXD0) U9.16(RXD0/DUPLEX)
ETHER_RXD1: U8.T2(ETHER_RXD1) U9.15(RXD1/PHYAD2)
ETHER_RXER: U8.M2(ETHER_RXER) U9.20(RXER/ISO)
ETHER_TXD0: U8.J2(ETHER_TXD0) U9.24(TXD0)
ETHER_TXD1: U8.H2(ETHER_TXD1) U9.25(TXD1)
ETHER_TXEN: U8.L2(ETHER_TXEN) U9.23(TXEN)
GND: ANT1.GND@0(GND) ANT1.GND@1(GND) ANT1.GND@2(GND) ANT1.GND@3(GND) ANT2.1(GND) ANT2.2(GND) C5.2 C11.2 C12.2 C13.2 C18.2 C19.2 C20.2 C24.2 C25.2 C26.2 C29.2 C30.2 C35.2 C36.2 C37.2 C40.2 C41.2 C43.2 C44.2 C45.2 C46.2 C53.2 C54.2 C58.2 C59.2 C60.2 C61.2 C62.2 C63.2 D1.2(VSS) D2.2 D8.2(VSS) D13.2 D15.2 D16.2 D17.2 D18.2 D19.2 D20.2 D21.2 D22.2 D23.2 D24.2 D25.2 D26.2 D27.2 D28.2 D31.2 D32.2 D33.2 D34.2 J3.6(GND) J3.10(GND) J3.11(GND) J3.12(GND) J3.13(GND) J5.8 J6.GND J6.GND2(GND) R13.2 R14.2 R22.1 R33.1 R34.1 R43.1 R44.1 R53.1 SHLD2.1 U4.P1(GND) U8.A3(RTC_XTALI) U8.A4(GND) U8.A7(GND) U8.A15(GND) U8.A16(GND) U8.A17(GND) U8.A21(GND) U8.A22(GND) U8.A23(GND) U8.AA13(GND) U8.AA14(GND) U8.AA15(GND) U8.AA16(GND) U8.AA17(GND) U8.AA18(GND) U8.AA19(GND) U8.AA20(GND) U8.AA21(GND) U8.AA22(GND) U8.AA23(GND) U8.AB2(GND) U8.AB3(GND) U8.AB4(GND) U8.AB5(GND) U8.AB6(GND) U8.AB7(GND) U8.AB8(GND) U8.AB13(GND) U8.AB14(GND) U8.AB15(GND) U8.AB16(GND) U8.AB17(GND) U8.AB18(GND) U8.AB19(GND) U8.AB20(GND) U8.AB21(GND) U8.AB22(GND) U8.AB23(GND) U8.AC13(GND) U8.AC15(GND) U8.AC18(GND) U8.AC19(GND) U8.AC21(GND) U8.AC22(GND) U8.AC23(GND) U8.B4(GND) U8.B5(GND) U8.B6(GND) U8.B7(GND) U8.B13(GND) U8.B17(GND) U8.B21(GND) U8.C4(GND) U8.C7(GND) U8.C15(GND) U8.C16(GND) U8.C17(GND) U8.C23(GND) U8.D2(GND) U8.D21(GND) U8.D22(GND) U8.D23(GND) U8.E2(GND) U8.E21(GND) U8.E22(GND) U8.E23(GND) U8.F21(GND) U8.F22(GND) U8.F23(GND) U8.G2(GND) U8.G21(GND) U8.G23(GND) U8.H21(GND) U8.H22(GND) U8.H23(GND) U8.J21(GND) U8.J22(GND) U8.J23(GND) U8.K2(GND) U8.K21(GND) U8.K22(GND) U8.K23(GND) U8.L21(GND) U8.L22(GND) U8.L23(GND) U8.M21(GND) U8.M22(GND) U8.N21(GND) U8.N22(GND) U8.P1(GND) U8.P2(GND) U8.P3(GND) U8.P21(GND) U8.P22(GND) U8.R3(GND) U8.R21(GND) U8.R22(GND) U8.T21(GND) U8.T22(GND) U8.T23(GND) U8.U2(GND) U8.U21(GND) U8.U22(GND) U8.U23(GND) U8.V21(GND) U8.V22(GND) U8.W21(GND) U8.W22(GND) U8.W23(GND) U8.Y2(GND) U8.Y21(GND) U8.Y22(GND) U8.Y23(GND) U9.1(GND) U9.GND U11.3(2A) U11.4(GND) U13.4(GND) U13.5(DIR) U14.4(GND) U15.4(GND) U15.5(DIR) U16.4(GND) U16.5(DIR) U16.6(2B) U17.4(GND) U18.4(GND) U18.5(DIR) ; also sheet 1
GND-ISO: C25.1 J2.7(GND) J2.8(GND) J2.S1(SHLD) J2.S2(SHLD) ; also sheet 1
GPIO_1: GPIO_1.1 U8.AA4(GPIO_1)
GPIO_2: GPIO_2.1 U8.L3(GPIO_2)
LED_PVT: U8.A14(GP_LED) ; also sheet 1
LED_RTK: U8.M3(GP_LED2) ; also sheet 1
LINK_MOSAIC: R6.2 R56.2 U9.30(LED0/NWAYEN)
LOG_LED: U8.B2(LOG_LED) ; also sheet 1
MOSAIC_!RST!: U8.A11(!RST!) ; also sheet 1
MOSAIC_CTS: U8.E1(COM1_CTS) U15.3(2A)
MOSAIC_CTS_I: D19.1 J5.3 U15.6(2B)
MOSAIC_EVENTA_1V8: U8.AC6(EVENTA) U13.2(1A)
MOSAIC_EVENTA_I: D15.1 J5.2 R43.2 U13.7(1B)
MOSAIC_EVENTB_1V8: U8.AC7(EVENTB) U13.3(2A)
MOSAIC_EVENTB_I: D13.1 J5.1 R44.2 U13.6(2B)
MOSAIC_LOG_BTN: U8.K3(LOG_BTN) U16.2(1A)
MOSAIC_LOG_BTN_I: D18.1 R23.2 U16.7(1B) ; also sheet 1
MOSAIC_PPSO: D16.1 U11.7(1B) ; also sheet 1
MOSAIC_PPSO_1V8: U8.AC8(PPS) U11.2(1A)
MOSAIC_RTS: U8.C1(COM1_RTS) U14.3(2A)
MOSAIC_RTS_O: D21.1 J5.4 U14.6(2B)
MOSAIC_RX: U8.B1(COM1_RX) U15.2(1A)
MOSAIC_RX_I: D20.1 J5.6 U15.7(1B)
MOSAIC_TX: U8.D1(COM1_TX) U14.2(1A)
MOSAIC_TX_O: D22.1 J5.5 U14.7(1B)
N$6: C37.1 R54.1 U4.P7(VREF2) U4.P8(EN)
N$8: J6.SHLD1(SHLD) J6.SHLD2(SHLD) J6.SHLD3(SHLD) J6.SHLD4(SHLD) SHLD2.2
N$9: R18.1 U8.AC3(SYNC)
N$13: C12.1 L2.2 L3.1
N$33: J6.B5(CC2) R33.2
N$34: J6.A5(CC1) R34.2
N$40: J2.14(GRN-) LINK2.1
N$41: J2.12(YLW-) SPEED2.1
N$42: I2C_IO.3 R_SCL_IO.2
N$43: I2C_IO.1 R_SDA_IO.2
N$142: R7.1 SPEED2.2
N$143: LINK2.2 R6.1
N$144: C29.1 R8.2 R9.2
N$145: C30.1 R10.2 R12.2
N$146: C35.1 C36.1 U9.2(VDDP)
N$147: C40.1 R13.1 R14.1 U9.10(REXT)
N$148: R15.1 U9.28(COL/CONFIG0)
PW+: J2.9(PW+) ; also sheet 1
PW-: J2.10(PW-) ; also sheet 1
RD+_MOSAIC: D1.1(IO1) J2.3(RD+) R12.1 U9.5(RX+)
RD-_MOSAIC: D1.3(IO2) J2.6(RD-) R10.1 U9.4(RX-)
RDY: RDY.1 U8.A12(MODULE_RDY)
REF: REF.1 U8.AC16(REF_OUT) U8.AC17(REF_IN)
SD_CLK: D32.1 J3.5(CLK/SCK) U8.AA1(SD_CLK)
SD_CMD: D33.1 J3.3(CMD/SDI) R46.1 U8.AB1(SD_CMD)
SD_DAT3: J3.2(DAT3/!CS!) R17.1
SD_DATA: D31.1 J3.7(DAT0/SDO) R47.1 U8.Y1(SD_DATA)
SPEED_MOSAIC: R7.2 R55.2 U9.31(LED1/SPEED)
TD+_MOSAIC: D1.6(IO4) J2.1(TD+) R8.1 U9.7(TX+)
TD-_MOSAIC: D1.4(IO3) J2.2(TD-) R9.1 U9.6(TX-)
V_USB_2: D8.5(VCC) J6.VBUS1(VBUS) J6.VBUS2(VBUS) VUSB2.1 ; also sheet 1
VANT: FB3.2 U8.P23(VANT) U8.R23(VANT)
VCCIO: C43.1 C44.1 C45.1 C59.1 I2C_IO.2 J5.7 R23.1 R54.2 U11.8(VCCB) U13.8(VCCB) U14.8(VCCB) U15.8(VCCB) U16.8(VCCB) U17.8(VCCB) U18.8(VCCB) ; also sheet 1
VDDA: C13.1 C24.1 C26.1 D1.5(VCC) FB1.2 J2.4(TCT) J2.5(RCT) U9.3(VDDA) VDDA.1
VIN+: J5.10 ; also sheet 1
VIN-: J5.9 ; also sheet 1
Unconnected: D8.4(IO3) D8.6(IO4) J3.1(DAT2) J3.8(DAT1) J3.9(DET) U8.A2(RTC_XTALO) U8.A9(RSVD_NC) U8.A10(ONOFF) U8.A13(RSVD_NC) U8.AA3(RSVD_NC) U8.AA5(RSVD_NC) U8.AA6(RSVD_NC) U8.AA7(RSVD_NC) U8.AA8(RSVD_NC) U8.AA9(RSVD_NC) U8.AA10(RSVD_NC) U8.AA11(RSVD_NC) U8.AA12(RSVD_NC) U8.AB9(RSVD_NC) U8.AB10(RSVD_NC) U8.AB11(RSVD_NC) U8.AB12(RSVD_NC) U8.AC1(RSVD_NC) U8.AC2(RSVD_NC) U8.AC5(RSVD_NC) U8.AC9(RSVD_NC) U8.AC10(RSVD_NC) U8.AC11(RSVD_NC) U8.AC12(RSVD_NC) U8.AC14(RSVD_NC) U8.B3(RSVD_NC) U8.B9(RSVD_NC) U8.B10(RSVD_NC) U8.B11(RSVD_NC) U8.B12(RSVD_NC) U8.B14(RSVD_NC) U8.B15(RSVD_NC) U8.B16(PMIC_ON_REQ) U8.B22(RSVD_NC) U8.B23(RSVD_NC) U8.C2(RSVD_NC) U8.C3(RSVD_NC) U8.C5(RSVD_NC) U8.C6(RSVD_NC) U8.C8(RSVD_NC) U8.C9(RSVD_NC) U8.C10(RSVD_NC) U8.C11(RSVD_NC) U8.C12(RSVD_NC) U8.C13(RSVD_NC) U8.C14(RSVD_NC) U8.C21(RSVD_NC) U8.C22(RSVD_NC) U8.F3(RSVD_NC) U8.G3(RSVD_NC) U8.G22(RSVD_NC) U8.H3(RSVD_NC) U8.J3(RSVD_NC) U8.N3(RSVD_NC) U8.R1(RSVD_NC) U8.T1(RSVD_NC) U8.T3(RSVD_NC) U8.U1(RSVD_NC) U8.U3(RSVD_NC) U8.V1(RSVD_NC) U8.V3(RSVD_NC) U8.W1(RSVD_NC) U8.W3(RSVD_NC) U8.Y3(RSVD_NC) U9.8(XO) U9.13(RXD3/PHYAD0) U9.14(RXD2/PHYAD1) U9.19(RXC) U9.21(INTRP) U9.22(TXC) U9.26(TXD2) U9.27(TXD3) U9.29(CRS/CONFIG1) U11.6(2B) U16.3(2A)

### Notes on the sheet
- Mosaic X5 | Mosaic IO Level Shifting
- 50Ω
- 50MHz
- 50Ω | 50Ω | 50Ω
- For future mosaic-H product:
  
  Populate: L2, L3, C12, ANT2
  Do Not Populate: R53
- 50Ω
- ESP32 IO Level Shifting
- microSD | Mosaic USB-C
- Open jumpers to
  disable pull-ups
- Open jumper to isolate shield
- Mag Jack - Mosaic | I/O Connector
- 50MHz
- Paul Clark
- v10
- Ethernet PHY - Mosaic

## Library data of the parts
1V8 2V8 3V3 3V3_SW 5V COM2_CTS COM2_RTS COM2_RX COM2_TX COM3_CTS COM3_RTS COM3_RX COM3_TX DTR ESP1 ESP2 ESP36 ESP39 GND GPIO_1 GPIO_2 RDY RDY1 REF RTS RX SCL2 SDA2 TP_BOOT TX VCCA VDDA VIN VPOE VUSB VUSB2 = SparkFun-Connectors:TEST-POINT: SparkFun Test Points
ANT1 = SparkFun-RF:ANTENNA-SMA-GROUNDED: SMA Antenna Connector w/ Ground; PROD_ID: CONN-08289
ANT2 = SparkFun-Connectors:U.FL2PIN: SMD Antenna Connector - U.FL
BOOT LOG_BTN RESET = SparkFun-Switches:MOMENTARY-SWITCH-SPST: Momentary Switch (Pushbutton) - SPST; PROD_ID: SWCH-13896
BOOT_SW BT LINK LINK2 LOAD LOG PVT PWR RESET_SW RTK SHLD1 SHLD2 SPEED SPEED2 WIFI = SparkFun-Jumpers:JUMPER-SMT_2_NC_TRACE: Normally closed trace jumper
C1 C3 C6 C8-C10 C14 C18 C33 C36 C46 C56 C60 C61 = SparkFun-Capacitors:2.2UF: 2.2µF ceramic capacitors; PROD_ID: CAP-07888
C2 C5 C7 C13 C15 C17 C19 C21-C23 C26-C31 C35 C37 C38 C41 C43 C44 C52 C53 C58 C59 C62 C63 = SparkFun-Capacitors:0.1UF: 0.1µF ceramic capacitors; PROD_ID: CAP-08604
C4 = SparkFun-Capacitors:10NF: 0.01uF/10nF/10,000pF ceramic capacitors; PROD_ID: CAP-00867
C11 C20 C24 C32 C39 C45 C54 C55 = SparkFun-Capacitors:10UF: 10.0µF ceramic capacitors; PROD_ID: CAP-11015
C12 = SparkFun-Capacitors:DNP: Do-Not-Populate capacitor
C16 C48 C57 = SparkFun-Capacitors:100UF-POLAR: 100µF polarized capacitors; PROD_ID: CAP-12547
C25 C42 = SparkFun-Capacitors:1.0NF/1000PF: 1nF/1,000pF ceramic capacitors; PROD_ID: CAP-16238
C34 C40 = SparkFun-Capacitors:100PF: 100pF/0.1nF ceramic capacitors; PROD_ID: CAP-07883
C47 C49-C51 C84 C85 = SparkFun-Capacitors:10UF: 10.0µF ceramic capacitors; PROD_ID: CAP-14259
C86 = SparkFun-Capacitors:47UF-POLAR: 47µF polarized capacitors; PROD_ID: CAP-10547
D1 D7 D8 D10 = SparkFun-DiscreteSemi:TVS_DIODE_ARRAY; PROD_ID: IC-13538
D2 D3 D13 D15-D34 = SparkFun-DiscreteSemi:PESD0402: ESD protection diode; DIGIKEY_PART: PESD0402-140CT-ND; MOUSE_PART: 650-PESD0402-140; PROD_ID: DIO-15359
D4-D6 D9 = SparkFun-DiscreteSemi:DIODE-SCHOTTKY: Schottky diode; PROD_ID: DIO-14072
D11 D12 = CBI_LED_TRIPLE-3MM:LED_TRIPLE-3MM_RIGHT-ANGLE_PTH: CBI LED Triple-3mm, Right Angle, PTH E.g.: LUMEX SSF-LXH340LYGID; PROD_ID: DIO-19990
D14 = SparkFun-DiscreteSemi:DIODE-SCHOTTKY: Schottky diode; PROD_ID: DIO-09886; VALUE: 3A/40V/500mV
ESP32_RF = SparkFun-RF:ANTENNA-SMA-GROUNDED: SMA Antenna Connector w/ Ground; PROD_ID: CONN-00827
F1 = SparkFun-Fuses:PPTC: Resettable Fuse PPTC; PROD_ID: RES-14313
FB1-FB3 = SparkFun-Coils:FERRITE_BEAD: Ferrite Bead (blocks, cores, rings, chokes, etc.); PROD_ID: NDUC-12579
FD1-FD4 = SparkFun-Aesthetics:FIDUCIAL: Fiducial Alignment Points
FRAME1 FRAME3 = SparkFun-Aesthetics:FRAME-LEDGER: Schematic Frame - Ledger
H1-H8 H10 = SparkFun-Hardware:STAND-OFF: Stand Off
I2C I2C_IO = SparkFun-Jumpers:JUMPER-SMT_3_2-NC_TRACE: Normally closed trace jumper (2 of 2 connections) This jumper has a trace between all three pads so they are normally closed (NC). Use a razor knife to open the connection(s). For best results follow the IPC guidelines for cutting traces: Cutout at least 0.063 mm (0.005 in). Remove all loose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
J1 J6 = SparkFun-Connectors:USB_C: USB Type C 16Pin Connector Super Speed pins not available on the 16-pin purely SMD connector so this part is best for USB 2.0 implementations. D1 and D2 are tied together enabling D+/- no matter which way the cable is plugged into the connector. The two channel configuration pins (CC1/2) are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; PROD_ID: CONN-14122
J2 J9 = SparkFun-Connectors:MAGJACK-POE: MAGJACK: RJ-45 with POE and LEDs This is a single port, RJ45 ethernet jacks with built in transformer (magnetics), PoE rectifier diodes, status LEDs, and shielding.; PROD_ID: CONN-16253
J3 = SparkFun-Connectors:MICRO-SD: microSD Socket for Transflash Various sockets for µSD. tDoc lines correctly indicate media card edge positions when inserting (unlocked, locked, depressed). NOTE: CD1 and CD2 are connected internally, and the default detect state of the socket is detect pin to ground. SparkFun Products: WAV Trigger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; PROD_ID: CONN-16110
J4 = SparkFun-Connectors:QWIIC_CONNECTOR: SparkFun I2C Standard Qwiic Connector An SMD 1mm pitch JST connector makes it easy and quick (get it? Qwiic?) to connect I2C devices to each other. The Qwiic system enables fast and solderless connection between popular platforms and various sensors and actuators. We carry 200mm, 100mm, 50mm, and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; PROD_ID: CONN-14483
J5 J13 = SparkFun-Connectors:CONN_10: Multi connection point. Often used as Generic Header-pin footprint for 0.1 inch spaced/style header connections On any of the 0.1 inch spaced packages, you can populate with these: Break Away Headers - Straight (PRT-00116) Break Away Male Headers - Right Angle (PRT-00553) Female Headers (PRT-00115)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; PROD_ID: CONN-17279; STOREFRONT: PRT-21328
J8 = SparkFun-Connectors:U.FL2PIN: SMD Antenna Connector - U.FL; PROD_ID: CONN-09193
L1 L4 = SparkFun-Coils:INDUCTOR: Inductors; PROD_ID: NDUC-14234
L2 L3 = SparkFun-Coils:DNP
LOGO1 = SparkFun-Aesthetics:SPECIAL_INSTRUCTIONS: Special Ordering/Production Instructions Alert
LOGO4 = SparkFun-Aesthetics:OSHW-LOGO: Open-Source Hardware (OSHW) Logo
LOGO5 = SparkFun-Aesthetics:SFE_LOGO_NAME: SparkFun Font Logo
LOGO6 = SparkFun-Aesthetics:SFE_LOGO_FLAME: SparkFun Flame Logo
MEAS PW+ PW- VIN+ VIN- = SparkFun-Jumpers:JUMPER-COMBO_2_NC_TRACE
MOSAIC_RST = SparkFun-Jumpers:JUMPER-COMBO_2_NO
Q1 = SparkFun-DiscreteSemi:TRANS_NPN_DUAL: Dual NPN Transistors in Single Package The MBT3904W1 puts two general purpose 3904 NPN transistors in a single package. Datasheet SparkFun Products: SparkFun ESP32 Thing; PROD_ID: TRANS-13337
R1 R2 R33 R34 = SparkFun-Resistors:5.1KOHM; PROD_ID: RES-12083
R3-R5 R15-R18 R22 R23 R29 R43 R44 R46-R50 = SparkFun-Resistors:10KOHM: 10kΩ resistor; PROD_ID: RES-00824
R6 R7 R19 R25-R27 = SparkFun-Resistors:1KOHM: 1kΩ resistor; PROD_ID: RES-07856
R8-R10 R12 R35 R40-R42 = SparkFun-Resistors:49.9OHM: 49.9Ω resistor; PROD_ID: RES-16237
R11 R13 R14 R24 = SparkFun-Resistors:13KOHM: 13kΩ resistor; PROD_ID: RES-14017
R20 R21 R55-R58 = SparkFun-Resistors:4.7KOHM: 4.7kΩ resistor; PROD_ID: RES-07857
R28 R36-R39 R59 = SparkFun-Resistors:470OHM: 470Ω resistor; PROD_ID: RES-07869
R30-R32 = SparkFun-Resistors:33OHM: 33Ω resistor; PROD_ID: RES-08270
R45 = SparkFun-Resistors:49.9OHM: 49.9Ω resistor; PROD_ID: RES-16252
R51-R53 = SparkFun-Resistors:0OHM: 0Ω resistor; PROD_ID: RES-08609
R54 = SparkFun-Resistors:200KOHM: 200kΩ resistor; PROD_ID: RES-09385
R_SCL R_SCL_IO R_SDA R_SDA_IO = SparkFun-Resistors:2.2KOHM: 2.2kΩ resistor; PROD_ID: RES-08272
T1 = SparkFun-Coils:TRANSFORMER: Small transformers; PROD_ID: COMP-19495
U1 = SparkFun-RF:ESP32-WROVER-E/IE: ESP32-WROVER-E/IE ESP32-WROVER-E uses the onboard antenna. ESP32-WROVER-IE has a u.FL antenna connector, but is otherwise the same as the -E. N16R8 has 16M Flash, 8M PSRAM; PROD_ID: IC-19265
U2 = SparkFun-IC-Comms:CH340C; PROD_ID: IC-14038
U3 U6 = SparkFun-IC-Power:AP7361C-33FGE: AP7361C 3.3V LDO Regulator; PROD_ID: VREG-14094
U4 = SparkFun-IC-Comms:PCA9306: Bidirectional I2C level shifter Not compatible with all available part number pinout schemes- DOUBLE CHECK!!! Variants PCA9306DC and PSOP-8 are EOL. If your part has VREF as pin 1 then this is your variant. VSSOP_8PIN is not EOL. Datasheet SparkFun Products SparkFun Inventor's Kit for RedBot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; PROD_ID: IC-14450
U7 U9 = Septentrio_mosaic-X5:KSZ8041NL; PROD_ID: IC-19428
U8 = Septentrio_mosaic-X5:MOSAIC-X5; PROD_ID: GPS-19395
U10 = SparkFun-IC-Power:POE_PSU: A special function Power Over Ethernet module with 5V or 12V output. Comes in an SMD package.; PROD_ID: IC-16251
U11 U13-U18 = 74LVC2T45DC:74LVC2T45: nexperia, 74LVC2T45, Dual supply translating transceiver, 3-state Source: product page, datasheet; PROD_ID: IC-19989
U12 = SparkFun-IC-Power:URB_YMD-15WR3: MORNSUN DC/DC Converter URB_YMD-15WR3 URB2405YMD-15WR3: Input 24V (9V-36V), Output 5.0V 3.0A; PROD_ID: COMP-19263
VCCIO = SparkFun-Switches:SWITCH-SPDT: Single Pole, Double Throw (SPDT) Switch Single-pole, double-throw (SPDT) switch. Variant Overview SMD-AYZ0202 Surface Mount DPDT Switch (COM-00597) Used on e.g. LilyPad Arduino USB - ATmega32U4 Board PTH-11.6X4.0MM SPDT Mini Power Switch (COM-00102) Used on e.g. SparkFun Simon Says - Through-Hole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; PROD_ID: SWCH-08179; SF_ID: COM-00597

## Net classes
2 3.3V: width 0.508 mm
3 RF_IN: width 0.35 mm, clearance 0.46 mm
4 USB: width 0.203 mm, clearance 0.127 mm
7 V_ZED: width 0.2 mm, clearance 0.2 mm
8 V_RF: width 0.2 mm
11 ZED_DIG: width 0.1 mm, clearance 0.1 mm

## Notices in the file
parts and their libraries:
SparkFun-Aesthetics: Licensing: Creative Commons ShareAlike 4.0 International - https://creativecommons.org/licenses/by-sa/4.0
SparkFun-Aesthetics: Released under the Creative Commons Attribution Share-Alike 4.0 License
SparkFun-Aesthetics: https://creativecommons.org/licenses/by-sa/4.0
